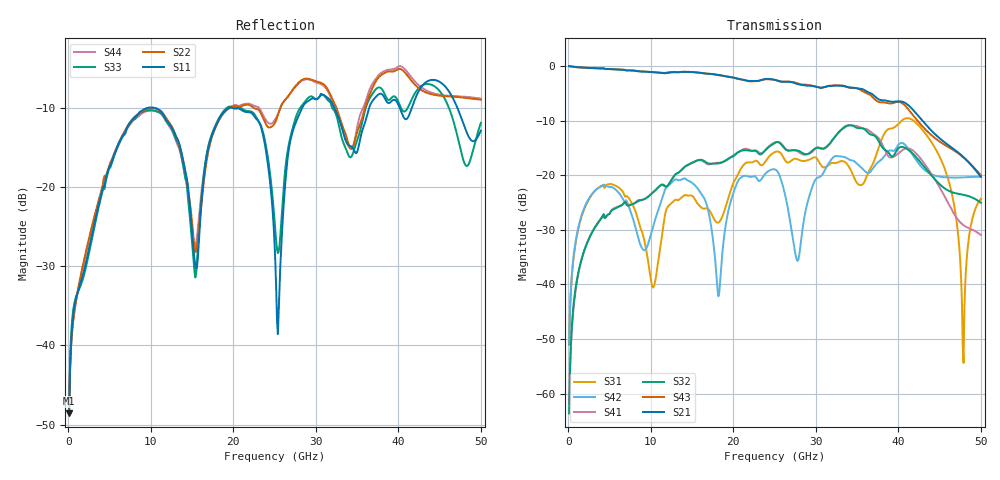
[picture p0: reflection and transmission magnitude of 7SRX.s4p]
! DAC39RF10ACK
! 256-pin FCBGA package
! Texas Instruments 8/20/2022
! Single-ended  S-parameters
! PORT#  PORT_NAME  NET_NAME
! PORT1:  xSRXN.DIEBUMP  xSRXN
! PORT2:  xSRXN.BGA  xSRXN
! PORT3:  xSRXP.DIEBUMP  xSRXP
! PORT4:  xSRXP.BGA  xSRXP
! Touchstone Ver. 1.0
! Number of ports is 4
# Hz	S	MA	R	50.000000
! SCATTERING PARAMETERS  :
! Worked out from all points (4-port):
!   500 points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, 100 MHz to 50 GHz, reference 50 ohm
!   strongest paths, dB at 100 MHz, 12.6 GHz, 25.1 GHz, 37.6 GHz, 50 GHz:
!     S21: 0.0, -1.2, -2.5, -6.1, -20.3
!     S43: 0.0, -1.1, -2.6, -6.6, -20.0
!     S32: -63.6, -20.6, -14.0, -13.7, -25.0
!     S41: -61.9, -20.6, -14.0, -13.2, -30.9
!     S42: -50.8, -21.2, -19.0, -17.5, -20.3
!     S31: -51.0, -25.0, -15.7, -15.0, -24.3
!   lowest |S11| = -48.6 dB at 100 MHz (marker M1), VSWR 1.01, Z = 50.3 + j0.208 ohm
!   |S11| at or under -10 dB: start of sweep to 9.457 GHz; 10.64 GHz to 19.4 GHz (8.756 GHz wide, 58.3 % of centre); 20 GHz to 28.32 GHz (8.317 GHz wide, 34.4 % of centre)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
1e8  0.003726 33.7  0.9959 -2.2  0.002942 85.0  0.0007232 -91.3
     0.9968 -2.1  0.004039 31.8  0.0007721 -96.6  0.003009 85.1
     0.002803 85.5  0.0006614 -88.9  0.004112 37.7  0.996 -2.2
     0.000804 -96.8  0.00288 85.8  0.9966 -2.2  0.003939 30.8
9e9  0.3072 -67.9  0.8878 -173.8  0.02919 -101.1  0.05931 85.3
     0.8882 -173.8  0.3024 -102.6  0.05847 84.2  0.02075 -139.6
     0.02937 -100.2  0.05978 84.1  0.3002 -69.4  0.8955 -174.3
     0.05932 84.7  0.02116 -136.6  0.8924 -174.2  0.295 -102.6
1.81e10  0.2593 -77.9  0.83 10.2  0.03798 -173.8  0.1288 -87.7
         0.8311 10.4  0.2553 -88.9  0.1289 -89.1  0.008873 7.0
         0.03674 -172.8  0.1281 -89.7  0.2632 -78.1  0.8273 9.8
         0.1301 -87.5  0.00876 4.1  0.8278 10.0  0.2622 -88.4
2.72e10  0.226 -48.1  0.7032 -165.3  0.1369 -144.3  0.1694 83.5
         0.7072 -165.1  0.4141 -120.3  0.1695 83.0  0.02745 -85.7
         0.1393 -144.2  0.1693 83.1  0.2376 -40.2  0.7119 -165.4
         0.1697 83.7  0.02646 -85.7  0.7122 -165.0  0.4132 -121.9
4.22e10  0.3801 -100.6  0.3311 -111.7  0.2855 -20.7  0.1492 119.7
         0.3649 -112.6  0.4357 -168.6  0.155 128.1  0.1345 31.3
         0.2992 -20.8  0.145 122.4  0.4072 -111.7  0.3401 -111.6
         0.1572 123.1  0.136 31.4  0.3237 -108.0  0.4564 -170.2
4.79e10  0.251 -144.9  0.135 161.4  0.004142 -117.9  0.05389 45.0
         0.1464 156.9  0.369 -166.7  0.06469 49.6  0.09907 33.2
         0.001913 42.6  0.06621 46.2  0.1473 -138.0  0.1354 159.0
         0.03484 40.8  0.09568 30.4  0.1454 171.9  0.3745 -168.1
5e10  0.2284 -104.1  0.08766 131.3  0.0564 -37.6  0.04755 12.6
      0.09677 126.8  0.358 -167.2  0.05312 16.0  0.101 28.5
      0.06105 -36.4  0.05592 10.8  0.2556 -87.7  0.08494 129.8
      0.02841 20.7  0.0969 27.4  0.1001 143.2  0.3645 -169.2
